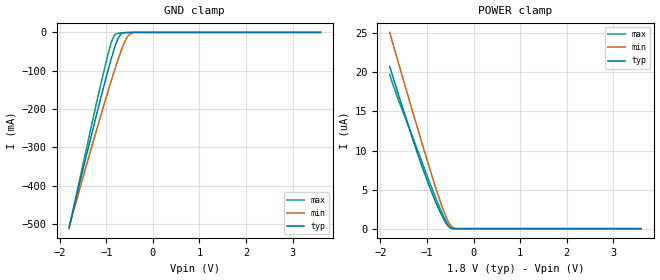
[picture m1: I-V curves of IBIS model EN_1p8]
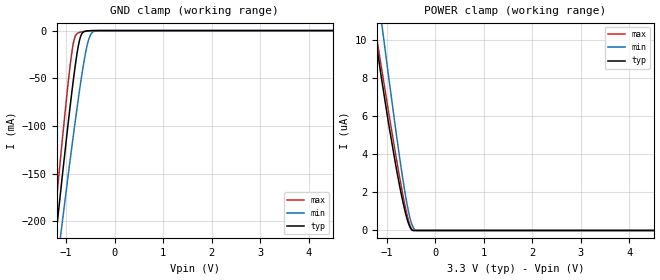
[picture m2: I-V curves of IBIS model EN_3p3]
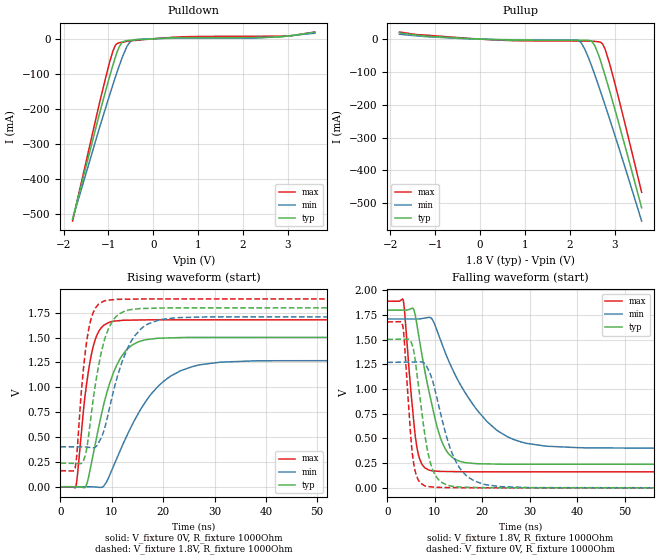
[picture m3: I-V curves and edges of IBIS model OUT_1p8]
|Texas Instruments Incorporated
| Marketing part#   Digital Voltage Range   Package-type   #pins
| LDC0851   1.71V - 3.46V   PWSON   8
[IBIS Ver]   4.1
[File name]   ldc0851.ibs
[File Rev]   1.0
[Date]   10/26/2015
[Source]
| Texas Instruments Incorporated.
| 12500 TI Blvd
| Dallas, TX -75243
[Notes]   Revision History:
| Rev 1.0: 10/26/2015
| - Initial version of the model
| - Model generated from simulations in TISPICE
| - C_comp although listed in numerical order of value are
|   obtained from varying PVT conditions. For PVT conditions for
|   each specific value refer the buffer description under
|   respective [Model]. IBIS model user is responsible for using
|   appropriate C_comp to simulate for Signal Integrity.
| - Warnings regarding combined Non-monotonicity of various models have been
|   reviewd and considered minor and can be ignored.
| - Model names with a trailing _1p8 contains the model for
|   1.8V operation.Model names with a trailing _3p3 contains the model
|   for 3.3V operation.
[Disclaimer]
| This model is designed as an aid for customers of Texas Instruments.
| TI and its licensors and suppliers make no warranties, either expressed
| or implied, with respect to this  model, including the warranties of
| merchantability or fitness for a particular purpose. The model is
| provided solely on an "as is" basis. The entire risk as to its quality
| and performance is with the customer.
[Copyright]
 (C) Copyright 2014 Texas Instruments Incorporated.All rights reserved.
|   Device
[Component] LDC0851
[Manufacturer]   TI
[Package]
|   typ   min   max
R_pkg   0.067   0.027   0.083
L_pkg   0.937nH   0.593nH   1.143nH
C_pkg   0.144pF   0.126pF   0.200pF
[Pin]  signal_name   model_name   R_pin   L_pin   C_pin
1   LCOM   NC   0   0   0
2   LSENSE   NC   0   0   0
3   LREF   NC   0   0   0
4   ADJ   NC   0   0   0
5   OUT   OUT   0   0   0
6   EN   EN   0   0   0
7   GND   GND   0   0   0
8   VDD   POWER   0   0   0
|   Model Selectors
[Model Selector]  OUT
OUT_3p3  output buffer at 3.3V operation.
OUT_1p8  output buffer at 1.8V operation.
[Model Selector]  EN
EN_3p3  input buffer at 3.3V operation.
EN_1p8  input buffer at 1.8V operation.
| Models and submodels in the file (4): EN_1p8 (Input), EN_3p3 (Input), OUT_1p8 (Output), OUT_3p3 (Output)
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|   Model
[Model]   EN_1p8
Model_type   Input
Vinl = 0.54
Vinh = 1.26
|   typ   min   max
C_comp   8.472pF   7.835pF   8.671pF
[Voltage Range]   1.8   1.71   1.89
[Temperature Range]   27   125   -40
[Power Clamp Reference]   1.8   1.71   1.89
[GND Clamp Reference]   0   0   0
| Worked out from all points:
|   GND clamp passes 1 mA (typ) near -0.63 V on its own axis
[GND Clamp]
|   Voltage   I(typ)   I(min)   I(max)
-1.8V     -507.5mA   -507.7mA   -512.1mA
-1.222V   -219.9mA   -259.5mA   -189.9mA
-1.001V   -115.7mA   -168.4mA   -74.16mA
-887.4mV  -65.79mA   -123.2mA   -23.99mA
-838.8mV  -46.04mA   -104.4mA   -9.817mA
-811.8mV  -35.82mA   -94.08mA   -5.576mA
-747mV    -15.1mA    -70.12mA   -2.296mA
-682.2mV  -3.658mA   -47.62mA   -1.356mA
-590.4mV  -470.3uA   -20.44mA   -568.1uA
-520.2mV  -139.6uA   -6.799mA   -215.2uA
-428.4mV  -17.41uA   -759.8uA   -26.26uA
3.6V      0A         0A         0A
[POWER Clamp]
|   Voltage   I(typ)   I(min)   I(max)
-1.8V     20.79uA    25.12uA    19.71uA
-1.714V   19.09uA    23.28uA    18.14uA
-1.595V   16.83uA    20.83uA    16.17uA
-1.292V   11.22uA    14.66uA    11.48uA
-1.103V   7.91uA     10.87uA    8.467uA
-941.4mV  5.298uA    7.685uA    5.906uA
-768.6mV  2.798uA    4.438uA    3.288uA
-628.2mV  1.076uA    2.058uA    1.372uA
-525.6mV  223.4nA    704.8nA    319.3nA
-444.6mV  0A         133.6nA    0A
-379.8mV  0A         0A         0A
3.6V      0A         0A         0A
|   Model
[Model]   EN_3p3
Model_type   Input
Vinl = 0.99
Vinh = 2.31
|   typ   min   max
C_comp   8.472pF   7.835pF   8.671pF
[Voltage Range]   3.3   3.14   3.46
[Temperature Range]   27   125   -40
[Power Clamp Reference]   3.3   3.14   3.46
[GND Clamp Reference]   0   0   0
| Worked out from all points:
|   GND clamp passes 1 mA (typ) near -0.63 V on its own axis
[GND Clamp]
|   Voltage   I(typ)   I(min)   I(max)
-3.3V     -1.281A    -1.179A    -1.373A
-1.28V    -248.2mA   -283.9mA   -221.6mA
-1.191V   -205mA     -246.6mA   -173.2mA
-1.102V   -162.6mA   -209.7mA   -125.8mA
-963.6mV  -98.9mA    -153.4mA   -56.31mA
-874.5mV  -60.41mA   -118.2mA   -19.52mA
-815.1mV  -37.03mA   -95.33mA   -5.957mA
-745.8mV  -14.79mA   -69.68mA   -2.271mA
-676.5mV  -3.163mA   -45.74mA   -1.294mA
-567.6mV  -317.9uA   -15.13mA   -431.6uA
-409.2mV  -10.13uA   -452.1uA   -14.43uA
6.6V      0A         0A         0A
[POWER Clamp]
|   Voltage   I(typ)   I(min)   I(max)
-3.3V     50.15uA    56.54uA    49.09uA
-1.3V     11.33uA    14.79uA    11.58uA
-1.162V   8.872uA    12uA       9.366uA
-1.112V   8.025uA    11.01uA    8.575uA
-963.6mV  5.61uA     8.09uA     6.223uA
-815.1mV  3.407uA    5.264uA    3.943uA
-706.2mV  1.953uA    3.31uA     2.368uA
-577.5mV  555.7nA    1.297uA    758.7nA
-478.5mV  10.14nA    280.8nA    34.68nA
-409.2mV  0A         6.597nA    0A
-260.7mV  0A         0A         0A
6.6V      0A         0A         0A
|   Model
[Model]   OUT_1p8
Model_type   Output
Polarity   Non-Inverting
Vmeas = 0.9
Vref = 0
Cref = 1pF
Rref = 100000
|   typ   min   max
C_comp   9.048pF   8.571pF   9.543pF
[Voltage Range]   1.8   1.71   1.89
[Temperature Range]   27   125   -40
[Pullup Reference]   1.8   1.71   1.89
[Pulldown Reference]   0   0   0
[Power Clamp Reference]   1.8   1.71   1.89
[GND Clamp Reference]   0   0   0
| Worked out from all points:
|   slope of the pulldown table from 0 to 0.27 V, typ, clamps not added: 155 ohm
|   slope of the pullup table from 0 to 0.27 V, typ, clamps not added: 195 ohm
|   falling waveform, V_fixture 1.8V, R_fixture 1000Ohm: 20-80 % time 4.1ns typ, 9.59ns min, 1.91ns max; typ from 1.8 V to 0.238 V
|   rising waveform, V_fixture 0V, R_fixture 1000Ohm: 20-80 % time 4.51ns typ, 8.43ns min, 2.37ns max; typ from 0 V to 1.5 V
|   rising waveform, V_fixture 1.8V, R_fixture 1000Ohm: 20-80 % time 3.06ns typ, 4.62ns min, 1.91ns max; typ from 0.238 V to 1.8 V
|   falling waveform, V_fixture 0V, R_fixture 1000Ohm: 20-80 % time 2.7ns typ, 4.67ns min, 1.52ns max; typ from 1.5 V to 0 V
[Pulldown]
|   Voltage   I(typ)   I(min)   I(max)
-1.8V     -514.9mA   -514.7mA   -520.1mA
-1.222V   -224.8mA   -263.6mA   -195.8mA
-1.012V   -124.8mA   -175.9mA   -85.15mA
-898.2mV  -74.38mA   -130.2mA   -34.52mA
-817.2mV  -41.91mA   -98.65mA   -14.77mA
-693mV    -9.832mA   -53.48mA   -9.569mA
-585mV    -5.157mA   -21.31mA   -7.378mA
-520.2mV  -4.336mA   -9.046mA   -6.3mA
-417.6mV  -3.344mA   -2.592mA   -4.89mA
689.4mV   3.166mA    1.63mA     5.72mA
2.812V    4.876mA    5.827mA    7.334mA
3.6V      18.72mA    15.8mA     19.21mA
[Pullup]
|   Voltage   I(typ)   I(min)   I(max)
-1.8V     18.9mA     14.76mA    21.58mA
311.4mV   -1.567mA   -976.1uA   -2.396mA
2.05V     -3.306mA   -2.016mA   -5.791mA
2.218V    -3.34mA    -7.021mA   -5.832mA
2.331V    -3.503mA   -30.1mA    -5.889mA
2.498V    -8.416mA   -86.92mA   -6.54mA
2.558V    -20.51mA   -109.6mA   -7.047mA
2.693V    -70.3mA    -163.4mA   -10.18mA
2.779V    -108.3mA   -198.9mA   -28.54mA
2.882V    -155.9mA   -241.7mA   -73.11mA
3.033V    -228.6mA   -305.9mA   -150.9mA
3.6V      -514.2mA   -554.5mA   -467mA
[Ramp]
R_load = 1000
|   typ   min   max
dV/dt_r   0.902124/4.50783e-09   0.762428/8.43863e-09   1.00791/2.37071e-09
dV/dt_f   0.937119/4.09884e-09   0.784713/9.59571e-09   1.03723/1.91049e-09
[Falling Waveform]
V_fixture = 1.8V
V_fixture_min = 1.71V
V_fixture_max = 1.89V
R_fixture = 1000Ohm
C_fixture = 0F
|   Time   V(typ)   V(min)   V(max)
0s        1.8V       1.71V      1.89V
3.339ns   1.8V       1.71V      1.903V
5.304ns   1.821V     1.71V      806.6mV
6.137ns   1.681V     1.71V      439.7mV
8.745ns   983.2mV    1.726V     180.8mV
11.14ns   514.4mV    1.507V     166.4mV
13.95ns   299.6mV    1.178V     164.4mV
20.99ns   242.4mV    671.9mV    162mV
28.07ns   239.2mV    466.4mV    162mV
100ns     238.1mV    402.1mV    161.3mV
[Rising Waveform]
V_fixture = 0V
V_fixture_min = 0V
V_fixture_max = 0V
R_fixture = 1000Ohm
C_fixture = 0F
|   Time   V(typ)   V(min)   V(max)
0s        -309.9nV   -2.262uV   -275.7nV
2.989ns   347.1uV    172.3uV    917.4uV
4.96ns    4.025mV    287.5uV    983mV
5.71ns    156.2mV    331.3uV    1.245V
6.802ns   436mV      -2.719mV   1.484V
9.474ns   1.022V     104mV      1.654V
12.69ns   1.366V     485.9mV    1.675V
17.44ns   1.484V     918.1mV    1.679V
25.94ns   1.502V     1.213V     1.679V
100ns     1.504V     1.271V     1.68V
[Rising Waveform]
V_fixture = 1.8V
V_fixture_min = 1.71V
V_fixture_max = 1.89V
R_fixture = 1000Ohm
C_fixture = 0F
|   Time   V(typ)   V(min)   V(max)
0s        238.1mV    402.1mV    161.3mV
2.878ns   234.5mV    402mV      192.6mV
4.554ns   271.9mV    401.6mV    1.223V
6.028ns   737.6mV    393.6mV    1.701V
8.433ns   1.451V     557.3mV    1.867V
10.35ns   1.684V     968.2mV    1.882V
13.15ns   1.777V     1.402V     1.887V
15.73ns   1.793V     1.591V     1.889V
19.06ns   1.797V     1.676V     1.889V
100ns     1.8V       1.71V      1.89V
[Falling Waveform]
|Gnd
V_fixture = 0V
V_fixture_min = 0V
V_fixture_max = 0V
R_fixture = 1000Ohm
C_fixture = 0F
|   Time   V(typ)   V(min)   V(max)
0s        1.504V     1.271V     1.68V
3.223ns   1.506V     1.273V     1.648V
5.435ns   1.416V     1.274V     286mV
6.431ns   1.084V     1.275V     88.14mV
7.88ns    545.8mV    1.258V     20.59mV
9.203ns   232.5mV    1.132V     10.14mV
10.84ns   80.27mV    831.3mV    4.617mV
14.44ns   12.57mV    266.2mV    2.143mV
19.93ns   2.593mV    41.72mV    833.5uV
100ns     -310nV     -226.3nV   -208.7nV
